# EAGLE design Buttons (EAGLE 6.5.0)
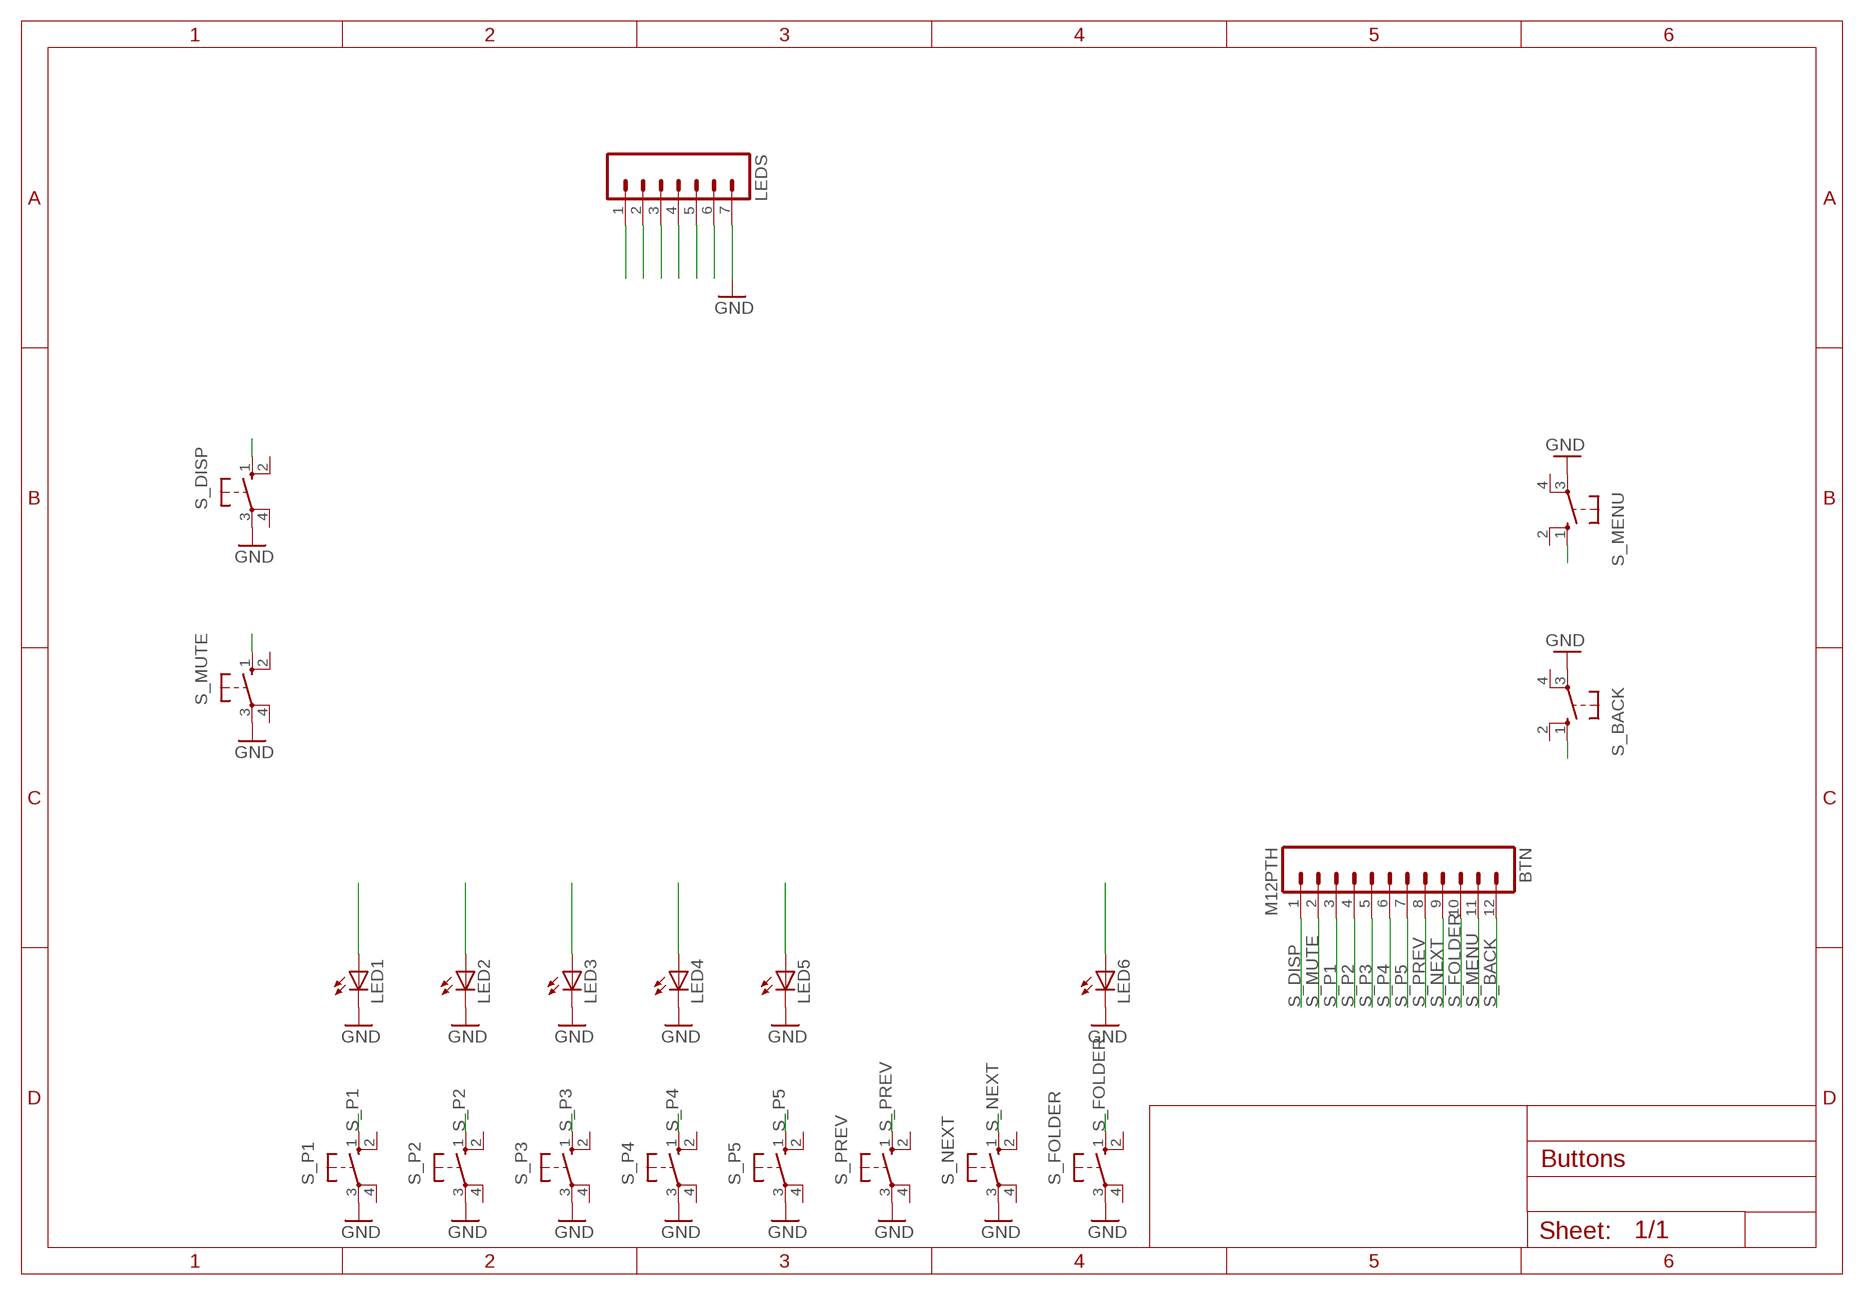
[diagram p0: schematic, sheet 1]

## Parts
BTN  M12PTH  [1X12]
LED1  LED3MM  [LED3MM]
LED2  LED3MM  [LED3MM]
LED3  LED3MM  [LED3MM]
LED4  LED3MM  [LED3MM]
LED5  LED3MM  [LED3MM]
LED6  LED3MM  [LED3MM]
LEDS  M07  [1X07]
S_BACK  10-XX  [B3F-10XX]
S_DISP  10-XX  [B3F-10XX]
S_FOLDER  10-XX  [B3F-10XX]
S_MENU  10-XX  [B3F-10XX]
S_MUTE  10-XX  [B3F-10XX]
S_NEXT  40-XX  [B3F-40XX]
S_P1  10-XX  [B3F-10XX]
S_P2  10-XX  [B3F-10XX]
S_P3  10-XX  [B3F-10XX]
S_P4  10-XX  [B3F-10XX]
S_P5  10-XX  [B3F-10XX]
S_PREV  40-XX  [B3F-40XX]

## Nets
GND [Ground]: LED1.K(C) LED2.K(C) LED3.K(C) LED4.K(C) LED5.K(C) LED6.K(C) LEDS.7 S_BACK.3(P) S_DISP.3(P) S_FOLDER.3(P) S_MENU.3(P) S_MUTE.3(P) S_NEXT.3(P) S_P1.3(P) S_P2.3(P) S_P3.3(P) S_P4.3(P) S_P5.3(P) S_PREV.3(P)
LED1: LED1.A LEDS.1
LED2: LED2.A LEDS.2
LED3: LED3.A LEDS.3
LED4: LED4.A LEDS.4
LED5: LED5.A LEDS.5
LED6: LED6.A LEDS.6
S_BACK: BTN.12 S_BACK.1(S)
S_DISP: BTN.1 S_DISP.1(S)
S_FOLDER: BTN.10 S_FOLDER.1(S)
S_MENU: BTN.11 S_MENU.1(S)
S_MUTE: BTN.2 S_MUTE.1(S)
S_NEXT: BTN.9 S_NEXT.1(S)
S_P1: BTN.3 S_P1.1(S)
S_P2: BTN.4 S_P2.1(S)
S_P3: BTN.5 S_P3.1(S)
S_P4: BTN.6 S_P4.1(S)
S_P5: BTN.7 S_P5.1(S)
S_PREV: BTN.8 S_PREV.1(S)
Unconnected: S_BACK.2(S1) S_BACK.4(P1) S_DISP.2(S1) S_DISP.4(P1) S_FOLDER.2(S1) S_FOLDER.4(P1) S_MENU.2(S1) S_MENU.4(P1) S_MUTE.2(S1) S_MUTE.4(P1) S_NEXT.2(S1) S_NEXT.4(P1) S_P1.2(S1) S_P1.4(P1) S_P2.2(S1) S_P2.4(P1) S_P3.2(S1) S_P3.4(P1) S_P4.2(S1) S_P4.4(P1) S_P5.2(S1) S_P5.4(P1) S_PREV.2(S1) S_PREV.4(P1)

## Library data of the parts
BTN = SparkFun-Connectors:M12: Header 12 Standard 12-pin 0.1" header. Use with straight break away headers (SKU : PRT-00116), right angle break away headers (PRT-00553), swiss pins (PRT-00743), machine pins (PRT-00117), and female headers (PRT-00115).
LED1-LED6 = led:LED: LED
LEDS = SparkFun-Connectors:M07: Header 7 Standard 7-pin 0.1" header. Use with straight break away headers (SKU : PRT-00116), right angle break away headers (PRT-00553), swiss pins (PRT-00743), machine pins (PRT-00117), and female headers (PRT-00115). NOTES ON THE VARIANTS LOCK and LOCK_LONGPADS... This footprint was designed to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
S_BACK S_DISP S_FOLDER S_MENU S_MUTE S_P1-S_P5 = switch-omron:10-XX: OMRON SWITCH; MPN: B3F-1000; OC_FARNELL: 176432; OC_NEWARK: 36M3542
S_NEXT S_PREV = switch-omron:40-XX: OMRON SWITCH; MF: OMRON COMPONENTS USA; MPN: B3F-4000; OC_FARNELL: 176434; OC_NEWARK: 36K3105

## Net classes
0 default: width 0.203 mm, drill 0.406 mm, clearance 0.203 mm
1 Power: width 0.61 mm, drill 0.711 mm, clearance 0.203 mm
2 Ground: width 0.508 mm, drill 0.711 mm, clearance 0.203 mm

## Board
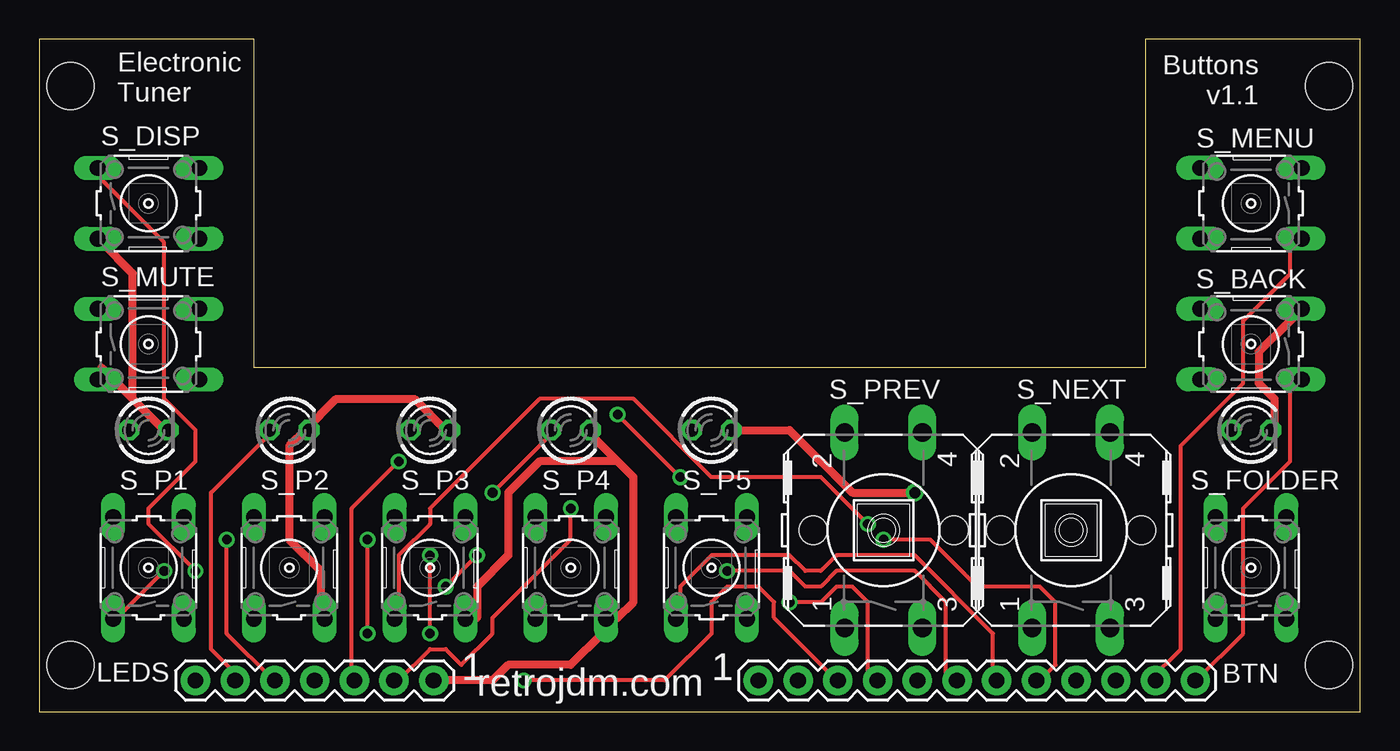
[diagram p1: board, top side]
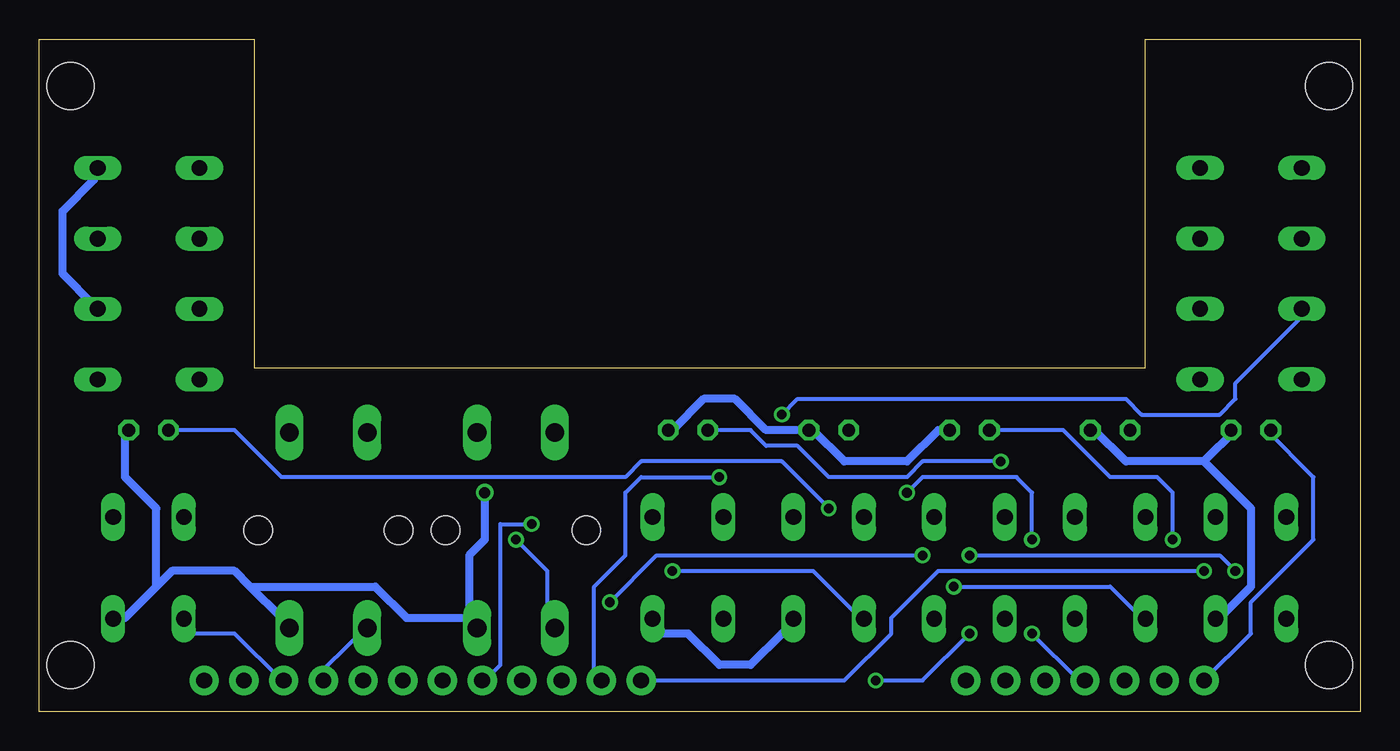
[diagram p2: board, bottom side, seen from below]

Size 84.5 x 43 mm. Coordinates in mm from the lower left corner, seen from the top.
Outline: 0,0 84.5,0 84.5,43 70.75,43 70.75,22 13.75,22 13.75,43 0,43 0,0
Copper layers (1*16): Top 0.035mm / dielectric 1.5mm / Bottom 0.035mm
Design rules "default *": minimum track width 10mil, minimum drill 24mil, track to track 0.2mm, track to pad 0.4mm, pad to pad 0.4mm, via to via 0.2mm, smd to smd 0.2mm, copper to edge 1mm, drill to drill 0.25mm, minimum pad ring 10mil, minimum via ring 8mil, stop-mask expansion 4mil, vias tented up to drill 0mil, thermal gap 10mil
Holes 3 mm at 2,40 2,3 82.5,40 82.5,3

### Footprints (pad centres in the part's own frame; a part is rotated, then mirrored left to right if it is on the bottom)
1X12 = drill 1.016 pad 1.88: 1 0,0; 2 2.54,0; 3 5.08,0; 4 7.62,0; 5 10.16,0; 6 12.7,0; 7 15.24,0; 8 17.78,0; 9 20.32,0; 10 22.86,0; 11 25.4,0; 12 27.94,0
LED3MM = drill 0.813 octagon: A -1.27,0; K 1.27,0
1X07 = drill 1.016 pad 1.88: 1 0,0; 2 2.54,0; 3 5.08,0; 4 7.62,0; 5 10.16,0; 6 12.7,0; 7 15.24,0
B3F-10XX = drill 1.016 long: 1 -3.251,2.261; 2 3.251,2.261; 3 -3.251,-2.261; 4 3.251,-2.261
B3F-40XX = drill 1.194 long: 1 -6.248,2.489; 2 6.248,2.489; 3 -6.248,-2.489; 4 6.248,-2.489 | hole 1.803: 0,-4.496; 0,4.496

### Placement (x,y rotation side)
BTN  46,2 0 top
LED1  7,18 0 top
LED2  16,18 0 top
LED3  25,18 0 top
LED4  34,18 0 top
LED5  43,18 0 top
LED6  77.5,18 0 top
LEDS  10,2 0 top
S_BACK  77.5,23.5 180 top
S_DISP  7,32.5 0 top
S_FOLDER  77.5,9.2 90 top
S_MENU  77.5,32.5 180 top
S_MUTE  7,23.5 0 top
S_NEXT  66,11.6 90 top
S_P1  7,9.2 90 top
S_P2  16,9.2 90 top
S_P3  25,9.2 90 top
S_P4  34,9.2 90 top
S_P5  43,9.2 90 top
S_PREV  54,11.6 90 top

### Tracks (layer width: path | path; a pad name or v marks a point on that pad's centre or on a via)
GND  (via drill 0.71)
  Top 0.508: LED6.K 79,18 79,20 78,21 78,23 80,25 S_BACK.3 | 37,16 38,15 38,7 37,6 S_P4.3 36,5 34,3 30,3 29,2 LEDS.7 | 37,16 35,18 LED4.K | 37,16 32,16 30,14 30,10 28,8 28,6 S_P3.3 | 6,20 4,22 S_MUTE.3 | 6,20 8,18 LED1.K | 17,18 19,20 24,20 26,18 LED3.K | 17,18 16,17 16,11 18,9 18,6 S_P2.3 | 17,18 LED2.K | 6,20 6,28 4,30 S_DISP.3 | v56,14 52,14 48,18 LED5.K 44,18
  Bottom 0.508: S_MENU.3 81,34 83,32 83,28 81,26 S_BACK.3 | 77,8 76,9 72,9 71,8 | 77,8 79,6 S_FOLDER.3 | 71,8 69,6 S_NEXT.3 | 57,6 61,6 63,8 71,8 | 77,8 77,13 79,15 79,18 LED6.K | LED5.K 44,18 42,20 40,20 38,18 LED4.K 35,18 33,16 29,16 27,18 LED3.K 26,18 | S_P5.3 45,5 43,5 41,3 39,3 37,5 S_P4.3 | 10,16 15,16 17,18 LED2.K | 10,16 8,18 LED1.K | 10,16 7,13 7,8 9,6 S_P1.3 | 57,6 57,10 56,11 v56,14 | 57,6 S_PREV.3
LED1
  Bottom 0.254: LEDS.1 7,5 7,7 3,11 3,15 6,18 LED1.A
LED2
  Top 0.254: LED2.A 15,18 11,14 11,4 13,2 LEDS.2
LED3  (via drill 0.61)
  Top 0.254: v12,11 12,5 15,2 LEDS.3
  Bottom 0.254: v12,11 12,14 13,15 16,15 19,18 LED3.A 24,18
LED4  (via drill 0.61)
  Top 0.254: v29,14 33,18 LED4.A | v21,5 v21,11
  Bottom 0.254: v29,14 28,15 22,15 21,14 v21,11 | v21,5 18,2 LEDS.4
LED5  (via drill 0.61)
  Top 0.254: v23,16 20,13 20,2 LEDS.5
  Bottom 0.254: v23,16 28,16 29,15 34,15 36,17 38,17 39,18 LED5.A 42,18
LED6  (via drill 0.61)
  Top 0.254: v34,13 34,11 29,6 29,5 27,3 26,4 25,4 23,2 LEDS.6
  Bottom 0.254: LED6.A 72,18 69,15 47,15 46,16 37,16 v34,13
S_BACK
  Top 0.254: S_BACK.1 80,21 80,16 77,13 77,5 74,2 BTN.12
S_DISP  (via drill 0.61)
  Top 0.254: v10,9 7,12 7,13 10,16 10,18 8,20 8,30 4,34 S_DISP.1
  Bottom 0.254: v10,9 27,9 30,6 30,5 33,2 BTN.1
S_FOLDER
  Bottom 0.254: S_FOLDER.1 75,5 72,5 69,2 BTN.10
S_MENU
  Top 0.254: S_MENU.1 80,30 80,28 77,25 77,21 73,17 73,4 71,2 BTN.11
S_MUTE  (via drill 0.61)
  Top 0.254: v41,15 v37,19
  Bottom 0.254: v37,19 36,20 15,20 14,19 9,19 8,20 8,21 4,25 S_MUTE.1 | v41,15 46,15 47,14 47,10 49,8 49,2 BTN.2
S_NEXT
  Bottom 0.254: S_NEXT.1 64,5 67,2 BTN.9
S_P1  (via drill 0.61)
  Top 0.254: v8,9 5,6 S_P1.1 | v25,5 v25,10 | v31,2 40,2 43,5 43,7 44,8 46,8 47,7 47,6 51,2 BTN.3
  Bottom 0.254: v8,9 9,10 v25,10 | v25,5 28,2 v31,2
S_P2  (via drill 0.61)
  Top 0.254: v28,10 v26,8 | v48,7 50,7 51,8 52,8 53,7 53,2 BTN.4
  Bottom 0.254: v26,8 16,8 14,6 S_P2.1 | v28,10 45,10 v48,7
S_P3  (via drill 0.61)
  Top 0.254: v53,12 50,15 43,15 38,20 32,20 25,13 25,12 23,10 23,6 S_P3.1
  Bottom 0.254: v53,12 55,12 55,3 56,2 BTN.5
S_P4  (via drill 0.61)
  Top 0.254: v44,9 48,9 49,8 50,8 51,9 56,9 58,7 58,2 BTN.6
  Bottom 0.254: v44,9 35,9 32,6 S_P4.1
S_P5
  Top 0.254: S_P5.1 41,6 41,8 43,10 48,10 49,9 50,9 51,10 56,10 61,5 61,2 BTN.7
S_PREV  (via drill 0.61)
  Top 0.254: v54,11 57,11 60,8 64,8 65,7 65,3 64,2 BTN.8
  Bottom 0.254: v54,11 52,9 52,6 S_PREV.1

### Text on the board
tNames: Buttons / v1.1 | Electronic / Tuner | 1 | 1 | retrojdm.com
